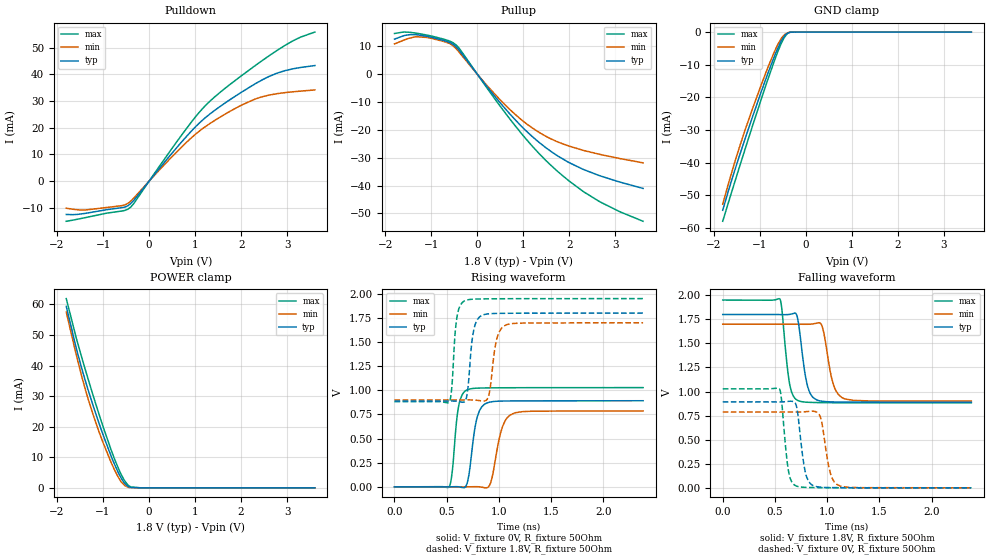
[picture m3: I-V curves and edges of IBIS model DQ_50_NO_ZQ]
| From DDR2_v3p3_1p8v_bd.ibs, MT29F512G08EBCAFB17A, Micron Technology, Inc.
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| MODEL DQ_50_NO_ZQ (50 Ohm Data I/O with no ODT, With No Cal)
[Model]   DQ_50_NO_ZQ
Model_type   I/O
Vinl = 650.000mV
Vinh = 1.150V
Vmeas = 900.000mV
Vref = 900.000mV
Cref = 0.0pF
Rref = 50.000Ohm
|   typ   min   max
|C_comp   1.200pF   1.100pF   1.300pF
C_comp_pullup   0.6000pF   0.5500pF   0.6500pF
C_comp_pulldown   0.6000pF   0.5500pF   0.6500pF
[Model Spec]
| Input threshold voltage corners
Vinl   0.6500V   0.6000V   0.7250V
Vinh   1.1500V   1.1000V   1.2250V
| Measurement voltage corners
Vmeas   0.9000V   0.8500V   0.9750V
| Timing spec test load voltage corners
Vref   0.9000V   0.8500V   0.9750V
| Dynamic Overshoot Parameters from ONFI4 Specification
D_overshoot_ampl_h   1.00   NA   NA
D_overshoot_ampl_l   1.00   NA   NA
D_overshoot_area_h   0.75n   NA   NA
D_overshoot_area_l   0.75n   NA   NA
[Receiver Thresholds]
Vth   =  0.900V
Vth_min  =  0.8820V
Vth_max  =  0.9180V
Vinh_ac  =  0.250V
Vinh_dc  =  0.125V
Vinl_ac  = -0.250V
Vinl_dc  = -0.125V
Tslew_ac =  5.000ns |Not specified, so set to high value
Threshold_sensitivity = 0.50
Reference_supply Pullup_ref
[Voltage Range]   1.8000V   1.7000V   1.9500V
[Pullup Reference]   1.8000V   1.7000V   1.9500V
| Junction Temperature (Ambient temp is 35C typ, 70C min, 0C max)
[Temperature Range]   50.0   85.0   0.0
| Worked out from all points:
|   slope of the pulldown table from 0 to 0.27 V, typ, clamps not added: 46.9 ohm
|   slope of the pullup table from 0 to 0.27 V, typ, clamps not added: 47.2 ohm
|   GND clamp passes 1 mA (typ) near -0.45 V on its own axis
|   POWER clamp passes 1 mA (typ) near -0.50 V on its own axis
|   falling waveform, V_fixture 1.8V, R_fixture 50Ohm: 20-80 % time 71.6ps typ, 83.6ps min, 61.1ps max; typ from 1.8 V to 0.889 V
|   rising waveform, V_fixture 0V, R_fixture 50Ohm: 20-80 % time 70.2ps typ, 90.2ps min, 54.6ps max; typ from 0 V to 0.892 V
|   rising waveform, V_fixture 1.8V, R_fixture 50Ohm: 20-80 % time 50.4ps typ, 60.5ps min, 41.9ps max; typ from 0.889 V to 1.8 V
|   falling waveform, V_fixture 0V, R_fixture 50Ohm: 20-80 % time 62.8ps typ, 72.8ps min, 54.5ps max; typ from 0.892 V to 0 V
[Pulldown]
|   Voltage   I(typ)   I(min)   I(max)
-1.8V     -12.5mA    -10.15mA   -15.05mA
-1.37V    -12.04mA   -10.79mA   -13.62mA
-598.1mV  -9.956mA   -9.21mA    -11.22mA
-450.2mV  -9.093mA   -8.215mA   -10.38mA
-331.7mV  -7.173mA   -6.308mA   -8.377mA
765.3mV   15.86mA    13.79mA    18.65mA
1.075V    21.52mA    18.55mA    25.5mA
1.326V    25.25mA    21.66mA    30.07mA
1.985V    33.13mA    28.32mA    39.26mA
2.603V    39.23mA    32.26mA    46.97mA
3.124V    42.12mA    33.51mA    52.61mA
3.6V      43.34mA    34.2mA     55.91mA
[GND Clamp]
|   Voltage   I(typ)   I(min)   I(max)
-1.8V     -54.56mA   -52.69mA   -57.93mA
-1.562V   -43.4mA    -40.96mA   -46.99mA
-1.429V   -37.59mA   -34.94mA   -41mA
-1.266V   -30.68mA   -28.04mA   -33.72mA
-952.2mV  -17.87mA   -15.76mA   -20.1mA
-822.5mV  -12.81mA   -10.99mA   -14.66mA
-599.8mV  -4.844mA   -3.701mA   -5.917mA
-525mV    -2.658mA   -1.9mA     -3.429mA
-462.3mV  -1.283mA   -878.8uA   -1.669mA
-397.8mV  -408.4uA   -316.9uA   -501uA
-322.2mV  -17.1uA    -69.38uA   0A
3.604V    0A         0A         0A
[Pullup]
|   Voltage   I(typ)   I(min)   I(max)
-1.8V     12.64mA    10.92mA    14.66mA
-1.494V   14.2mA     12.91mA    15.13mA
-1.102V   13.66mA    13.25mA    14.12mA
-599.8mV  11.4mA     11.06mA    11.92mA
-462.3mV  9.867mA    9.209mA    10.58mA
576.6mV   -11.83mA   -10.55mA   -13.26mA
962.5mV   -18.77mA   -16.42mA   -21.38mA
1.353V    -24.65mA   -21.01mA   -28.72mA
1.765V    -29.56mA   -24.44mA   -35.23mA
2.338V    -34.45mA   -27.51mA   -42.55mA
3.076V    -38.66mA   -30.23mA   -49.27mA
3.6V      -41.04mA   -31.85mA   -52.85mA
[POWER Clamp]
|   Voltage   I(typ)   I(min)   I(max)
-1.8V     59.37mA    57.52mA    61.9mA
-1.591V   46.25mA    44.06mA    49.53mA
-1.436V   37.64mA    34.94mA    41.24mA
-1.215V   26.85mA    23.86mA    30.17mA
-1.095V   21.42mA    18.62mA    24.4mA
-824.2mV  10.35mA    8.287mA    12.39mA
-672.9mV  5.125mA    3.568mA    6.58mA
-599.8mV  3.04mA     1.802mA    4.182mA
-462.1mV  554.9uA    243.4uA    940.1uA
-396mV    138.1uA    64.45uA    266.2uA
-178.2mV  714nA      206.6nA    547.3nA
3.604V    0A         0A         0A
[Ramp]
R_load = 50
|   typ   min   max
dV/dt_r 5.3523E-01/7.0119E-11   4.7192E-01/9.0196E-11   6.1686E-01/5.4437E-11
dV/dt_f 5.4672E-01/7.1389E-11   4.7943E-01/8.3486E-11   6.4049E-01/6.0993E-11
[Falling Waveform]
V_fixture = 1.8V
V_fixture_min = 1.7V
V_fixture_max = 1.95V
R_fixture = 50Ohm
C_fixture = 0F
|   Time   V(typ)   V(min)   V(max)
0s        1.8V       1.7V       1.95V
548ps     1.799V     1.7V       1.96V
640ps     1.801V     1.7V       1.082V
726ps     1.705V     1.699V     903.9mV
810ps     1.065V     1.699V     888.6mV
900ps     913.3mV    1.71V      885.6mV
952ps     899.1mV    1.676V     884.7mV
1.06ns    892.1mV    1.071V     883.8mV
1.138ns   890.8mV    939.2mV    883.5mV
2.38ns    888.8mV    900.9mV    882.5mV
[Rising Waveform]
V_fixture = 0V
V_fixture_min = 0V
V_fixture_max = 0V
R_fixture = 50Ohm
C_fixture = 0F
|   Time   V(typ)   V(min)   V(max)
0s        85.56uV    160.6uV    23.59uV
522ps     345.8uV    112.6uV    -2.465mV
552ps     1.183mV    108uV      151.2mV
614ps     831.9uV    67.47uV    835.2mV
700ps     56.53mV    481.8uV    1.007V
786ps     696.4mV    1.827mV    1.022V
888ps     870.3mV    -8mV       1.025V
1.034ns   888.8mV    623.4mV    1.026V
1.11ns    890mV      745.6mV    1.027V
2.38ns    892.1mV    786.7mV    1.028V
[Rising Waveform]
V_fixture = 1.8V
V_fixture_min = 1.7V
V_fixture_max = 1.95V
R_fixture = 50Ohm
C_fixture = 0F
|   Time   V(typ)   V(min)   V(max)
0s        888.7mV    900.8mV    882.5mV
522ps     888.9mV    900.7mV    875.7mV
548ps     889.1mV    900.7mV    1.022V
598ps     886.5mV    900.6mV    1.758V
676ps     888.6mV    900.7mV    1.929V
760ps     1.631V     899.6mV    1.944V
846ps     1.781V     888.8mV    1.947V
900ps     1.792V     939mV      1.948V
1.05ns    1.798V     1.667V     1.949V
2.38ns    1.8V       1.7V       1.95V
[Falling Waveform]
|Gnd
V_fixture = 0V
V_fixture_min = 0V
V_fixture_max = 0V
R_fixture = 50Ohm
C_fixture = 0F
|   Time   V(typ)   V(min)   V(max)
0s        892.2mV    786.8mV    1.028V
542ps     891.7mV    786.9mV    1.028V
630ps     898.2mV    787mV      172.8mV
702ps     862.4mV    786.4mV    20.31mV
786ps     187.6mV    789.8mV    5.158mV
862ps     25.26mV    795.8mV    3.092mV
938ps     6.294mV    725.1mV    2.035mV
1.034ns   2.557mV    139.9mV    1.419mV
1.126ns   1.644mV    17.88mV    1.084mV
2.38ns    171.2uV    281.9uV    79.04uV
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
